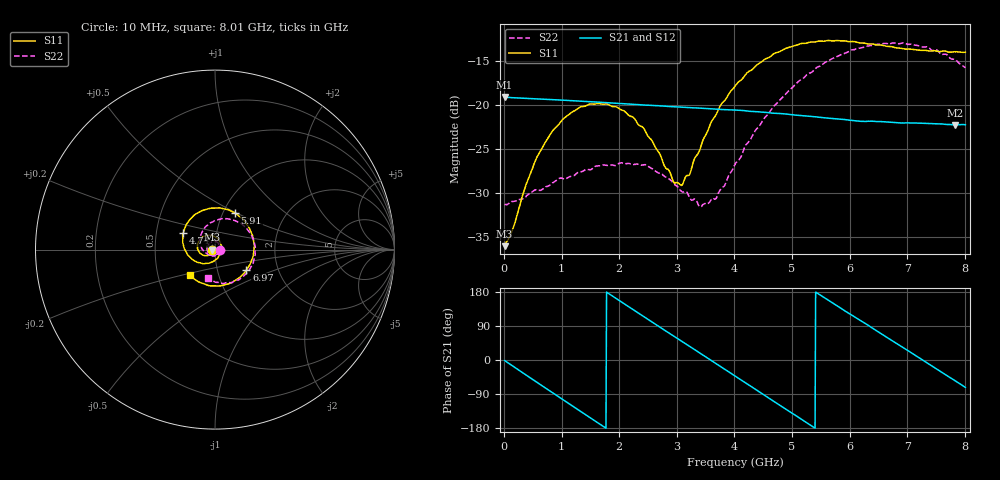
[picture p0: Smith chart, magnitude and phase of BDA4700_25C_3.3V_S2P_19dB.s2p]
!Agilent Technologies,E5071B,MY42404982,A.09.10
!Date: Mon Oct 20 18:11:01 2025
!Data & Calibration Information:
!Freq	S11:SOLT2(ON)	S21:SOLT2(ON)	S12:SOLT2(ON)	S22:SOLT2(ON)
# Hz S RI R 50
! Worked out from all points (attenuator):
!   801 points, 10 MHz to 8.01 GHz, reference 50 ohm
!   highest |S21| = -19.08 dB at 10 MHz (marker M1); lowest = -22.3 dB at 7.83 GHz (marker M2)
!   lowest |S11| = -36.1 dB at 10 MHz (marker M3), VSWR 1.03, Z = 48.5 - j0.114 ohm
!   |S11| at or under -10 dB: start of sweep to end of sweep
!   |S22| runs from -31.6 to -12.9 dB; largest |S21 - S12| = 0.0013
!   S11 on the Smith chart (normalised r, x): 10 MHz: 0.97, -0.00; 4.74 GHz: 0.69, +0.13; 5.91 GHz: 1.14, +0.49; 6.97 GHz: 1.38, -0.33; 8.01 GHz: 0.73, -0.22
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1e7  -0.0156 -0.00118  0.1111 -0.00241  0.1111 -0.00249  0.0271 -0.00088
1.5e8  -0.0169 -0.00996  0.106 -0.03  0.106 -0.03  0.0272 -0.00745
6e8  -0.0406 -0.0334  0.0513 -0.0955  0.0513 -0.0955  0.0127 -0.03
1.01e9  -0.0787 -0.0242  -0.0247 -0.1039  -0.0247 -0.1038  -0.0166 -0.0345
1.35e9  -0.0978 0.00762  -0.0779 -0.0708  -0.0779 -0.0709  -0.0381 -0.017
2.08e9  -0.0489 0.079  -0.0873 0.0524  -0.0873 0.0524  -0.0282 0.0368
2.42e9  -0.00229 0.0741  -0.0425 0.0907  -0.0426 0.0906  -0.00122 0.0455
2.68e9  0.0255 0.0479  0.00114 0.0991  0.000953 0.0991  0.0173 0.0372
2.95e9  0.0353 0.00823  0.0449 0.0869  0.0448 0.0867  0.029 0.0205
3.09e9  0.0322 -0.0136  0.0643 0.073  0.0637 0.0735  0.0308 0.00861
3.4e9  0.00342 -0.0555  0.0913 0.0301  0.0914 0.0301  0.0217 -0.015
3.54e9  -0.0181 -0.0693  0.0953 0.00728  0.0953 0.00723  0.0126 -0.0245
3.69e9  -0.0461 -0.0763  0.0933 -0.0171  0.0933 -0.0174  -0.00129 -0.0296
4.01e9  -0.1108 -0.0641  0.0695 -0.0629  0.0695 -0.0627  -0.0358 -0.0283
4.74e9  -0.1777 0.0911  -0.0375 -0.0815  -0.037 -0.0818  -0.0833 0.06
5.35e9  -0.0628 0.2201  -0.0858 -0.00761  -0.0857 -0.00814  -0.0141 0.1541
5.91e9  0.1121 0.2037  -0.0536 0.063  -0.0538 0.0627  0.1171 0.1586
6.68e9  0.2148 -0.0219  0.0441 0.0666  0.0443 0.0667  0.2235 -0.00896
6.97e9  0.1751 -0.1135  0.0693 0.0382  0.0694 0.0378  0.2068 -0.0875
7.44e9  0.039 -0.2001  0.0751 -0.0229  0.0751 -0.0228  0.107 -0.1743
7.83e9  -0.0914 -0.1799  0.0448 -0.0628  0.0448 -0.063  0.00263 -0.1819
8.01e9  -0.1402 -0.1434  0.0234 -0.0736  0.0237 -0.0736  -0.0404 -0.1582
